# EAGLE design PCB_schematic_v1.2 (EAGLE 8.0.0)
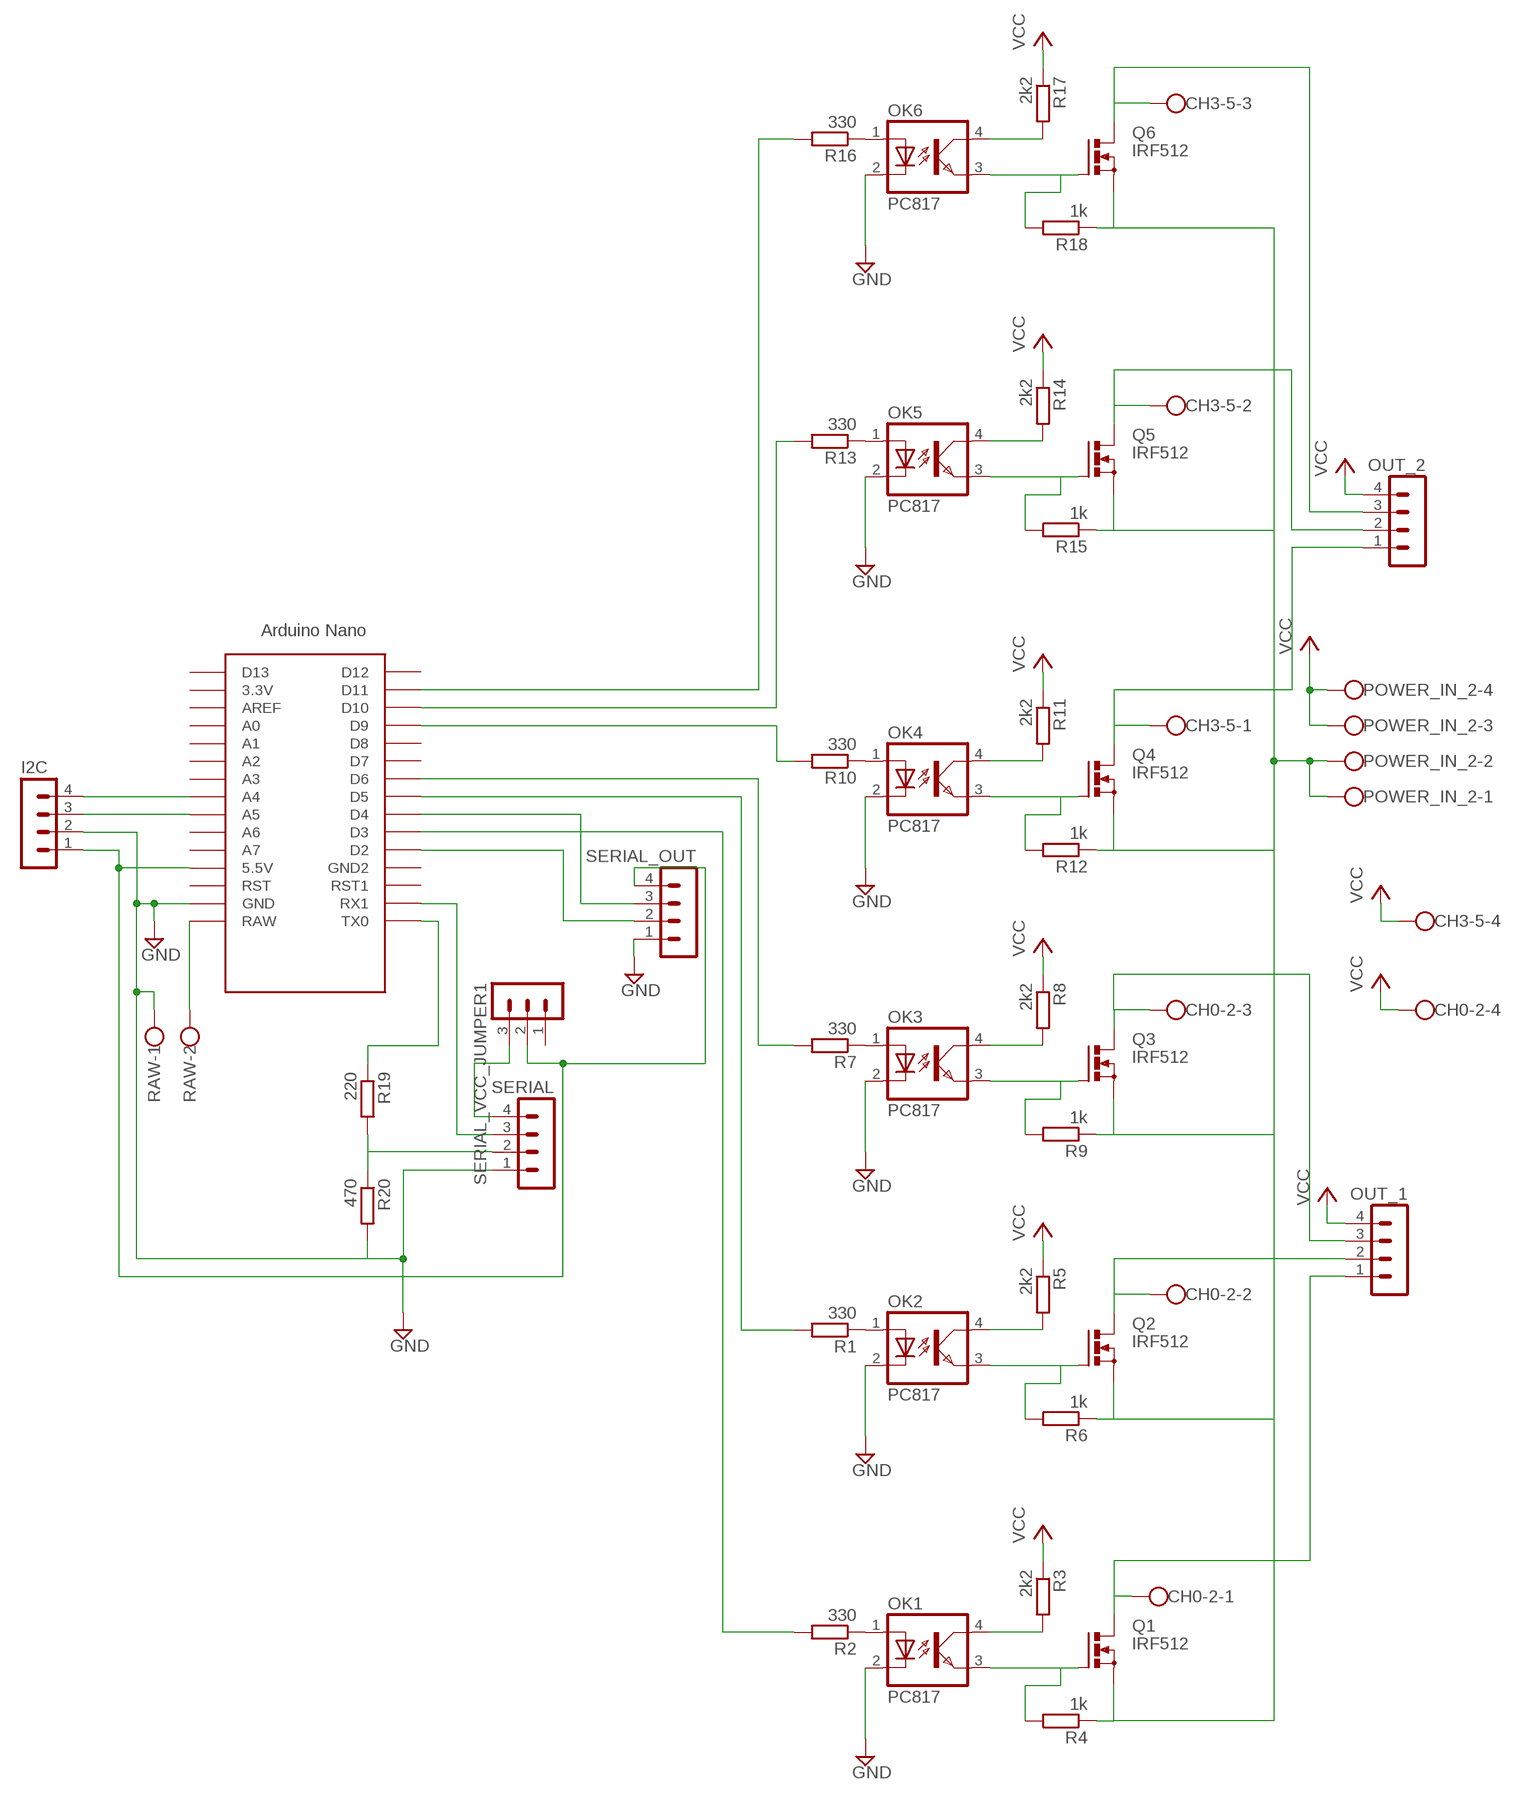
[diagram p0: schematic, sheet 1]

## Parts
CH0-2  W237-4  [W237-4]
CH3-5  W237-4  [W237-4]
I2C  MA04-1  [MA04-1]
OK1  PC817  [DIL04]
OK2  PC817  [DIL04]
OK3  PC817  [DIL04]
OK4  PC817  [DIL04]
OK5  PC817  [DIL04]
OK6  PC817  [DIL04]
OUT_1  MA04-1  [MA04-1]
OUT_2  MA04-1  [MA04-1]
POWER_IN_2  W237-4  [W237-4]
Q1  IRF512  [TO220BV]
Q2  IRF512  [TO220BV]
Q3  IRF512  [TO220BV]
Q4  IRF512  [TO220BV]
Q5  IRF512  [TO220BV]
Q6  IRF512  [TO220BV]
R1  330  R-EU_0207/10  [0207/10]
R2  330  R-EU_0207/10  [0207/10]
R3  2k2  R-EU_0207/10  [0207/10]
R4  1k  R-EU_0207/10  [0207/10]
R5  2k2  R-EU_0207/10  [0207/10]
R6  1k  R-EU_0207/10  [0207/10]
R7  330  R-EU_0207/10  [0207/10]
R8  2k2  R-EU_0207/10  [0207/10]
R9  1k  R-EU_0207/10  [0207/10]
R10  330  R-EU_0207/10  [0207/10]
R11  2k2  R-EU_0207/10  [0207/10]
R12  1k  R-EU_0207/10  [0207/10]
R13  330  R-EU_0207/10  [0207/10]
R14  2k2  R-EU_0207/10  [0207/10]
R15  1k  R-EU_0207/10  [0207/10]
R16  330  R-EU_0207/10  [0207/10]
R17  2k2  R-EU_0207/10  [0207/10]
R18  1k  R-EU_0207/10  [0207/10]
R19  220  R-EU_0207/10  [0207/10]
R20  470  R-EU_0207/10  [0207/10]
RAW  W237-102  [W237-102]
SERIAL  MA04-1  [MA04-1]
SERIAL_OUT  MA04-1  [MA04-1]
SERIAL_VCC_JUMPER1  MA03-1  [MA03-1]
U$1  NANO  [NANO]

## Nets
EXT_GND: POWER_IN_2.1 POWER_IN_2.2 Q1.S Q2.S Q3.S Q4.S Q5.S Q6.S R4.1 R6.1 R9.1 R12.1 R15.1 R18.1
EXT_VCC_12V: CH0-2.4 CH3-5.4 OUT_1.4 OUT_2.4 R3.1 R5.1 R8.1 R11.1 R14.1 R17.1 ; supply symbol labelled VCC
FET0_GATE: OK1.3(EMIT) Q1.G R4.2
FET0_GATE1: OK2.3(EMIT) Q2.G R6.2
FET0_GATE2: OK3.3(EMIT) Q3.G R9.2
FET0_GATE3: OK4.3(EMIT) Q4.G R12.2
FET0_GATE4: OK5.3(EMIT) Q5.G R15.2
FET0_GATE5: OK6.3(EMIT) Q6.G R18.2
GND: I2C.2 OK1.2(C) OK2.2(C) OK3.2(C) OK4.2(C) OK5.2(C) OK6.2(C) R20.2 RAW.1 SERIAL.1 SERIAL_OUT.1 U$1.GND
IC_PWM_OUT_0: R2.2 U$1.D3
IC_PWM_OUT_0_BASE: OK1.1(A) R2.1
IC_PWM_OUT_0_BASE1: OK2.1(A) R1.1
IC_PWM_OUT_0_BASE2: OK3.1(A) R7.1
IC_PWM_OUT_0_BASE3: OK4.1(A) R10.1
IC_PWM_OUT_0_BASE4: OK5.1(A) R13.1
IC_PWM_OUT_0_BASE5: OK6.1(A) R16.1
IC_PWM_OUT_1: R1.2 U$1.D5
IC_PWM_OUT_2: R7.2 U$1.D6
IC_PWM_OUT_3: R10.2 U$1.D9
IC_PWM_OUT_4: R13.2 U$1.D10
IC_PWM_OUT_5: R16.2 U$1.D11
IC_VCC_5V: I2C.1 SERIAL_OUT.4 SERIAL_VCC_JUMPER1.2 U$1.5V(5.5V)
N$1: OK1.4(COL) R3.2
N$3: OK2.4(COL) R5.2
N$5: OK3.4(COL) R8.2
N$7: OK4.4(COL) R11.2
N$9: OK5.4(COL) R14.2
N$11: OK6.4(COL) R17.2
N$28: SERIAL_OUT.3 U$1.D4
N$29: SERIAL_OUT.2 U$1.D2
OUTPUT_0: CH0-2.1 OUT_1.1 Q1.D
OUTPUT_1: CH0-2.2 OUT_1.2 Q2.D
OUTPUT_2: CH0-2.3 OUT_1.3 Q3.D
OUTPUT_3: CH3-5.1 OUT_2.1 Q4.D
OUTPUT_4: CH3-5.2 OUT_2.2 Q5.D
OUTPUT_5: CH3-5.3 OUT_2.3 Q6.D
RAW_INPUT: RAW.2 U$1.RAW
RX: SERIAL.3 U$1.RX1
SCL: I2C.3 U$1.A5
SDA: I2C.4 U$1.A4
SERIAL_VCC: SERIAL.4 SERIAL_VCC_JUMPER1.3
TX_3,3V: R19.2 R20.1 SERIAL.2
TX_5V: R19.1 U$1.TX0
VCC: POWER_IN_2.3 POWER_IN_2.4
Unconnected: SERIAL_VCC_JUMPER1.1 U$1.3.3V U$1.A0 U$1.A1 U$1.A2 U$1.A3 U$1.A6 U$1.A7 U$1.AREF U$1.D7 U$1.D8 U$1.D12 U$1.D13 U$1.GND1(GND2) U$1.ICSP1 U$1.ICSP2 U$1.ICSP3 U$1.ICSP4 U$1.ICSP5 U$1.ICSP6 U$1.RST U$1.RST1

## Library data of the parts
CH0-2 CH3-5 POWER_IN_2 = con-wago-500:W237-4: WAGO SCREW CLAMP; OC_FARNELL: unknown; OC_NEWARK: unknown
I2C OUT_1 OUT_2 SERIAL SERIAL_OUT = con-lstb:MA04-1: PIN HEADER; OC_FARNELL: unknown; OC_NEWARK: unknown
OK1-OK6 = optocoupler:PC817: SHARP OPTO COUPLER; MPN: PC817X4J000F; OC_FARNELL: 9707727; OC_NEWARK: 97K7059
Q1-Q6 = transistor-power:IRF512: N-CHANNEL MOS FET
R1-R20 = rcl:R-EU_: RESISTOR, European symbol
RAW = con-wago-500:W237-102: WAGO SCREW CLAMP; MPN: 237-102; OC_FARNELL: unknown; OC_NEWARK: 70K9898
SERIAL_VCC_JUMPER1 = con-lstb:MA03-1: PIN HEADER; OC_FARNELL: unknown; OC_NEWARK: unknown
U$1 = Arduino-clone:NANO: Arduino Nano

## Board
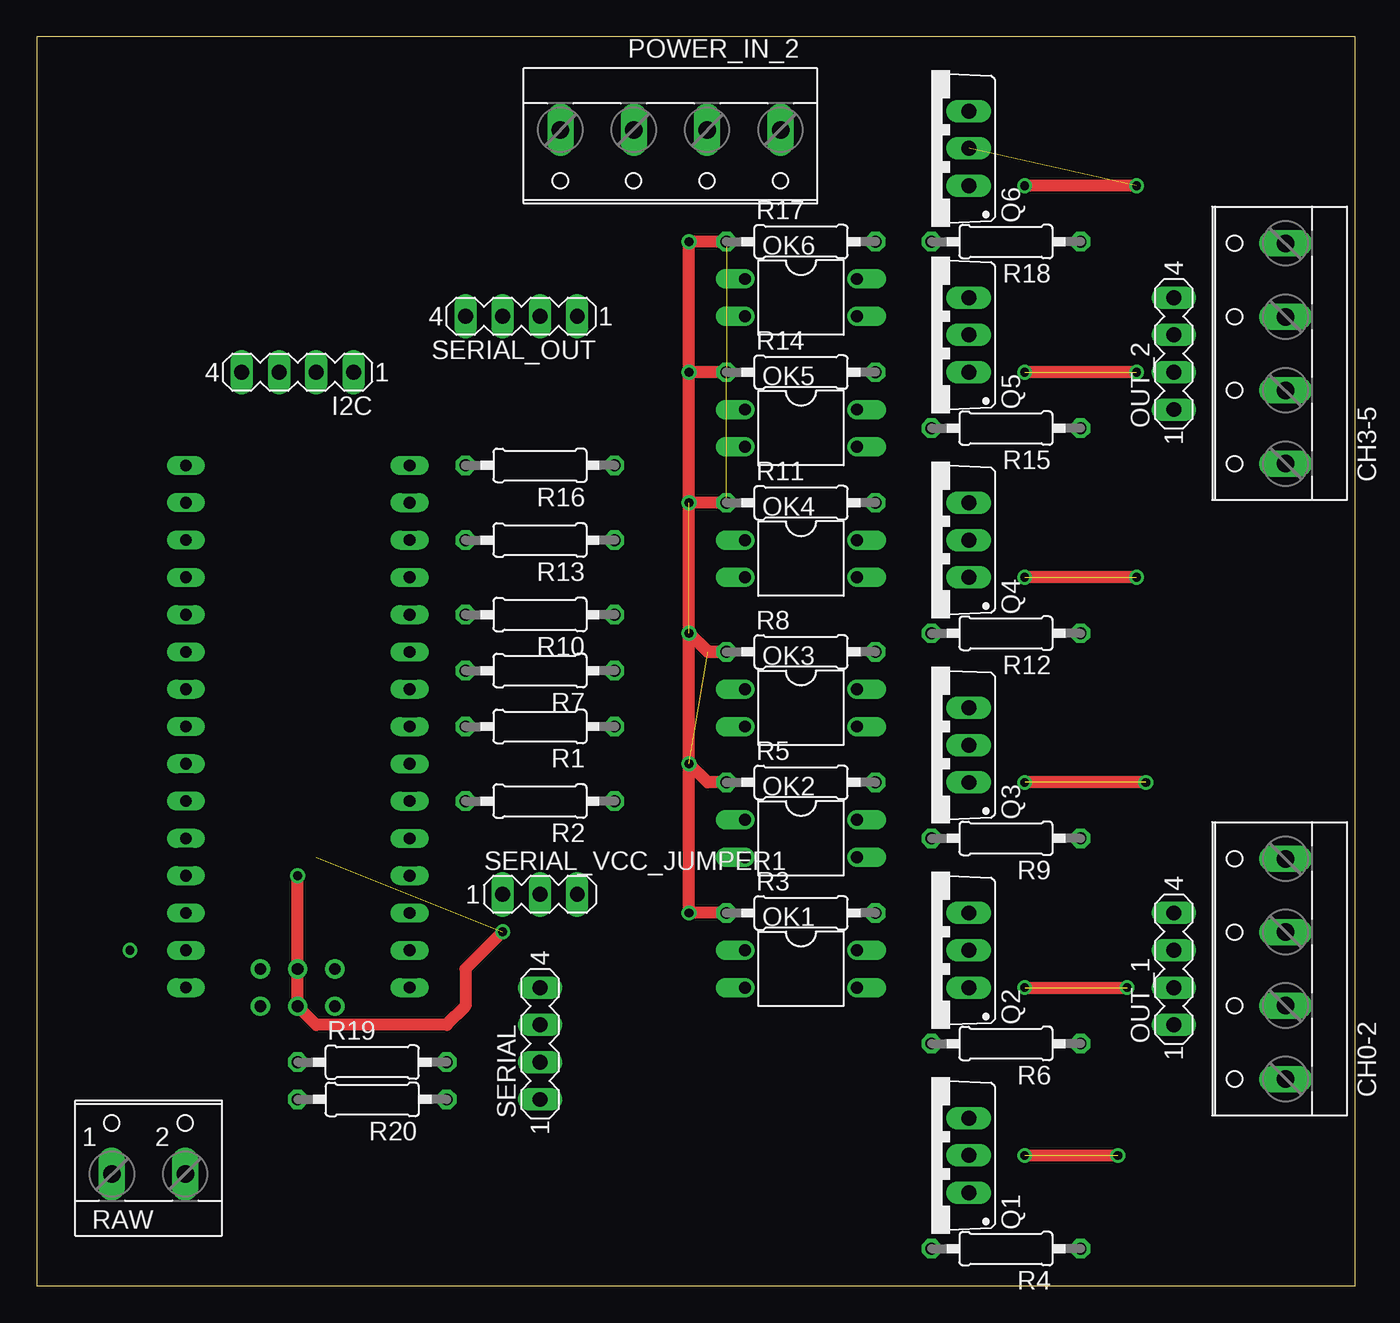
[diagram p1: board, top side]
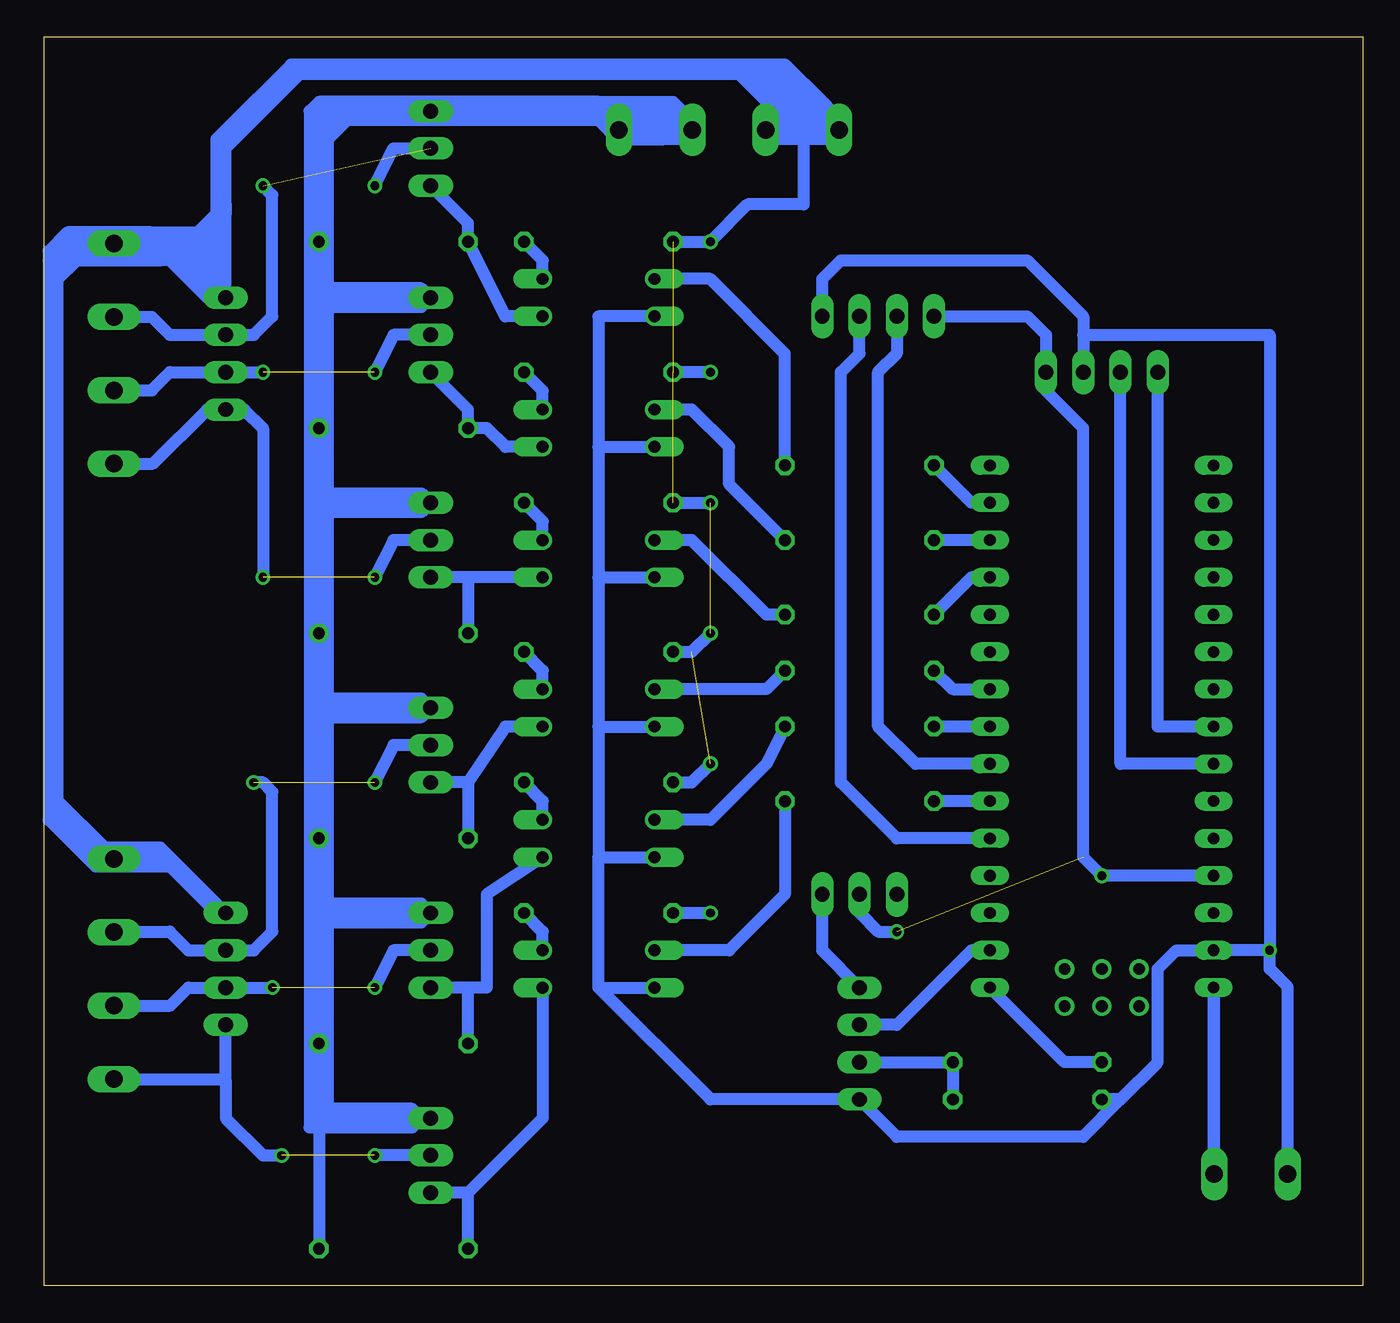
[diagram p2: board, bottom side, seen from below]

Size 89.84 x 85.08 mm. Coordinates in mm from the lower left corner, seen from the top.
Outline: 0,0 89.84,0 89.84,85.08 0,85.08 0,0
Copper layers (1*16): Top 0.035mm / dielectric 1.5mm / Bottom 0.035mm
Design rules "default": minimum track width 10mil, minimum drill 24mil, track to track 8mil, track to pad 8mil, pad to pad 8mil, via to via 8mil, smd to smd 8mil, copper to edge 40mil, drill to drill 8mil, minimum pad ring 10mil, minimum via ring 8mil, stop-mask expansion 4mil, vias tented up to drill 0mil, thermal gap 10mil

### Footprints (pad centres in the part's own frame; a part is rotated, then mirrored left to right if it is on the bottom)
W237-4 = drill 1.194 long: 1 -7.5,-1.27; 2 -2.5,-1.27; 3 2.5,-1.27; 4 7.5,-1.27
MA04-1 = drill 1.016 long: 1 -3.81,0; 2 -1.27,0; 3 1.27,0; 4 3.81,0
DIL04 = drill 0.813 offset: 1 -1.27,-3.81; 2 1.27,-3.81; 3 1.27,3.81; 4 -1.27,3.81
TO220BV = drill 1.016 long: D 0,-2.54; G -2.54,-2.54; S 2.54,-2.54
0207/10 = drill 0.813 octagon: 1 -5.08,0; 2 5.08,0
W237-102 = drill 1.194 long: 1 -2.5,-1.27; 2 2.5,-1.27
MA03-1 = drill 1.016 long: 1 -2.54,0; 2 0,0; 3 2.54,0
NANO = drill 0.8 long: 3.3V -10.16,24.13; 5V -10.16,-1.27; A0 -10.16,19.05; A1 -10.16,16.51; A2 -10.16,13.97; A3 -10.16,11.43; A4 -10.16,8.89; A5 -10.16,6.35; A6 -10.16,3.81; A7 -10.16,1.27; AREF -10.16,21.59; D2 5.08,1.27; D3 5.08,3.81; D4 5.08,6.35; D5 5.08,8.89; D6 5.08,11.43; D7 5.08,13.97; D8 5.08,16.51; D9 5.08,19.05; D10 5.08,21.59; D11 5.08,24.13; D12 5.08,26.67; D13 -10.16,26.67; GND -10.16,-6.35; GND1 5.08,-1.27; RAW -10.16,-8.89; RST -10.16,-3.81; RST1 5.08,-3.81; RX1 5.08,-6.35; TX0 5.08,-8.89 | drill 0.8: ICSP1 -5.08,-10.16; ICSP2 -5.08,-7.62; ICSP3 -2.54,-10.16; ICSP4 -2.54,-7.62; ICSP5 0,-10.16; ICSP6 0,-7.62

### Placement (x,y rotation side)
CH0-2  83.82,21.59 90 top
CH3-5  83.82,63.5 90 top
I2C  17.78,62.23 180 top
OK1  52.07,21.59 270 top
OK2  52.07,30.48 270 top
OK3  52.07,39.37 270 top
OK4  52.07,49.53 270 top
OK5  52.07,58.42 270 top
OK6  52.07,67.31 270 top
OUT_1  77.47,21.59 90 top
OUT_2  77.47,63.5 90 top
POWER_IN_2  43.18,77.47 180 top
Q1  60.96,8.89 90 top
Q2  60.96,22.86 90 top
Q3  60.96,36.83 90 top
Q4  60.96,50.8 90 top
Q5  60.96,64.77 90 top
Q6  60.96,77.47 90 top
R1  34.29,38.1 180 top
R2  34.29,33.02 180 top
R3  52.07,25.4 0 top
R4  66.04,2.54 180 top
R5  52.07,34.29 0 top
R6  66.04,16.51 180 top
R7  34.29,41.91 180 top
R8  52.07,43.18 0 top
R9  66.04,30.48 180 top
R10  34.29,45.72 180 top
R11  52.07,53.34 0 top
R12  66.04,44.45 180 top
R13  34.29,50.8 180 top
R14  52.07,62.23 0 top
R15  66.04,58.42 180 top
R16  34.29,55.88 180 top
R17  52.07,71.12 0 top
R18  66.04,71.12 180 top
R19  22.86,15.24 0 top
R20  22.86,12.7 180 top
RAW  7.62,8.89 0 top
SERIAL  34.29,16.51 90 top
SERIAL_OUT  33.02,66.04 180 top
SERIAL_VCC_JUMPER1  34.29,26.67 0 top
U$1  20.32,29.21 0 top

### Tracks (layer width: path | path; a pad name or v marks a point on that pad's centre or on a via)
EXT_GND
  Bottom 0.813: 71.12,11.43 R4.1 | 71.12,11.43 R6.1 71.12,25.4 | 71.12,25.4 R9.1 71.12,39.37 | 71.12,39.37 R12.1 | 71.12,53.34 R15.1 | 71.12,53.34 R12.1 | 71.12,66.67 R15.1 | 71.12,79.38 71.12,80.01 69.22,80.01 | 71.12,78.74 71.12,78.11 | 71.12,78.11 R18.1 71.12,67.31 | Q5.S 71.12,67.31 | Q4.S 71.12,53.34 | Q2.S 71.12,25.4 | Q1.S 64.14,11.43 | 64.14,11.43 71.12,11.43 | Q6.S 52.07,80.01 50.8,78.7 POWER_IN_2.2 POWER_IN_2.1 | Q6.S 69.22,80.01 | R15.1 R12.1 | Q3.S 71.12,39.37 | 69.22,79.38 52.07,79.38 50.8,78.11 50.16,78.11 | 69.22,79.38 70.48,79.38 | 70.48,79.38 71.12,78.74 | 71.12,78.74 71.12,79.38 | 71.12,79.38 70.48,79.38 | 50.16,78.11 50.16,78.74 52.07,80.64 | 52.07,80.64 71.12,80.64 71.75,80.01 71.75,10.79 64.77,10.79 64.14,11.43 | 64.14,11.43 64.77,12.06 70.48,12.06 70.48,24.77 | 70.48,26.04 70.48,38.73 | 70.48,40.01 70.48,52.7 | 70.48,53.98 70.48,78.11 69.22,79.38 | 70.48,52.7 64.14,52.7 Q4.S | 70.48,52.7 70.48,53.98 | 70.48,53.98 64.14,53.98 Q4.S | Q3.S 64.14,40.01 70.48,40.01 | 70.48,40.01 70.48,38.73 | 70.48,38.73 64.14,38.73 Q3.S | Q2.S 64.14,26.04 70.48,26.04 | 70.48,26.04 70.48,24.77 | 70.48,24.77 64.14,24.77 Q2.S | Q5.S 64.14,67.94 70.48,67.94 71.12,67.31 | 71.12,67.31 71.12,66.67 | 71.12,66.67 64.14,66.67 Q5.S | 71.12,78.11 69.22,80.01 | Q6.S 52.7,80.01 52.07,80.64 | 52.07,80.64 46.99,80.64 45.72,79.38 45.72,78.11 47.62,78.11 | 50.16,78.11 47.62,78.11 | 47.62,78.11 46.35,79.38 | 46.35,79.38 46.99,79.38 | 46.99,79.38 47.62,80.01 | 47.62,80.01 46.99,80.01 46.35,79.38 | 46.99,79.38 50.16,79.38 50.8,80.01 47.62,80.01
EXT_VCC_12V  (4 unrouted)
  Top 0.813: R14.1 44.45,62.23 | R17.1 44.45,71.12 | R11.1 44.45,53.34 | R5.1 45.72,34.29 44.45,35.56 44.45,25.4 R3.1 | R8.1 45.72,43.18 44.45,44.45
  Bottom 0.813: OUT_1.4 81.16,29.09 CH0-2.4 86.24,29.09 88.9,31.75 88.9,32.38 | 81.28,69.85 82.43,71 CH3-5.4 85.21,71.12 87.63,71.12 | 81.28,69.85 79.38,67.94 | 78.74,67.31 OUT_2.4 77.47,73.03 | R17.1 44.45,71.12 41.91,73.66 38.1,73.66 38.1,80.64 | R11.1 44.45,53.34 | R8.1 45.72,43.18 44.45,44.45 | R5.1 45.72,34.29 44.45,35.56 | R3.1 44.45,25.4 | 77.47,73.66 77.47,77.47 72.39,82.55 42.55,82.55 | 41.91,82.55 41.27,82.55 | 41.27,82.55 40.64,82.55 | 40.01,82.55 39.37,82.55 38.1,81.28 38.1,80.64 | 88.9,33.02 88.9,68.58 | 88.9,68.58 88.9,69.85 88.27,70.48 | 40.64,80.01 40.64,79.38 | 40.64,79.38 38.73,79.38 | 38.73,79.38 35.56,79.38 | 35.56,79.38 35.56,78.11 40.64,78.11 40.64,79.38 | 38.73,79.38 38.73,80.64 40.64,82.55 | 40.64,82.55 40.01,82.55 | 40.01,82.55 38.1,80.64 | 38.1,80.64 36.83,80.64 | 36.83,80.64 36.2,80.01 | 36.2,80.01 35.56,79.38 | 36.83,80.64 39.37,83.19 72.39,83.19 | 72.39,83.19 73.03,83.19 77.47,78.74 | 77.47,78.74 78.11,78.11 78.11,69.22 | 78.11,69.22 78.74,68.58 | 78.74,68.58 79.38,68.58 | 79.38,68.58 80.01,69.22 | 80.01,69.22 81.92,71.12 | 81.92,71.12 82.55,71.75 | 82.55,71.75 88.27,71.75 89.53,70.48 89.53,69.85 | 89.53,69.85 89.53,31.75 86.36,28.57 81.28,28.57 78.11,25.4 OUT_1.4 | OUT_1.4 81.92,29.84 85.72,29.84 88.9,33.02 | 88.9,33.02 88.9,32.38 | 88.9,32.38 85.72,29.21 | 88.27,70.48 87.63,71.12 | 87.63,71.12 88.27,71.12 89.53,69.85 | 89.53,69.85 87.63,69.85 | 87.63,69.85 81.92,69.85 | 81.28,69.85 81.92,69.85 | 81.92,69.85 82.55,70.48 88.27,70.48 | 79.38,68.58 79.38,67.94 | 79.38,67.94 78.74,67.31 | 78.74,67.31 78.11,67.94 78.11,68.58 | 78.11,69.22 78.11,68.58 | 78.11,68.58 78.74,67.94 | 88.9,68.58 87.63,69.85 | 82.55,71.75 79.38,71.75 77.47,73.66
  Bottom 0.813: 77.47,73.66 77.47,73.03 | 77.47,73.03 79.38,71.12 81.28,71.12 | 81.92,71.12 81.28,71.12 | 81.28,71.12 80.64,70.48 | 80.64,70.48 78.74,68.58 | 78.74,68.58 78.74,69.85 | 78.74,69.85 78.74,71.12 80.01,71.12 80.64,70.48 | 80.64,70.48 79.38,70.48 78.74,69.85 | 78.74,69.85 79.38,69.85 80.01,69.22 | 80.01,69.22 79.38,69.22 78.74,69.85 | 77.47,78.74 77.47,78.11 72.39,83.19 | 36.2,80.01 40.64,80.01 | 40.64,80.01 40.64,80.64 42.55,82.55 | 42.55,82.55 41.91,82.55 | 41.91,82.55 40.01,80.64 39.37,80.64 41.27,82.55
FET0_GATE
  Bottom 0.813: R4.2 60.96,6.35 | OK1.3 55.88,11.43 60.96,6.35 | 60.96,6.35 Q1.G
FET0_GATE1
  Bottom 0.813: R6.2 60.96,20.32 | OK2.3 59.69,26.67 59.69,20.32 60.96,20.32 | 60.96,20.32 Q2.G
FET0_GATE2
  Bottom 0.813: 60.96,34.29 Q3.G | OK3.3 58.42,38.1 60.96,34.29 | 60.96,34.29 R9.2
FET0_GATE3
  Bottom 0.813: 60.96,48.26 R12.2 | 60.96,48.26 Q4.G | OK4.3 60.96,48.26
FET0_GATE4
  Bottom 0.813: Q5.G 60.96,59.69 R15.2 59.69,58.42 58.42,57.15 OK5.3
FET0_GATE5
  Bottom 0.813: Q6.G 60.96,72.39 R18.2 58.42,66.04 OK6.3
GND  (via drill 0.6)
  Bottom 0.813: OK6.2 52.07,66.04 52.07,57.15 | 52.07,57.15 OK5.2 | 52.07,57.15 52.07,48.26 | 52.07,48.26 OK4.2 | 52.07,48.26 52.07,38.1 | 52.07,38.1 OK3.2 | 52.07,38.1 52.07,29.21 | 52.07,29.21 OK2.2 | 52.07,20.32 52.07,29.21 | 52.07,20.32 OK1.2 | 52.07,20.32 44.45,12.7 SERIAL.1 31.75,10.16 19.05,10.16 16.51,12.7 | 16.51,12.7 R20.2 | 16.51,12.7 13.97,15.24 13.97,21.59 12.7,22.86 U$1.GND v6.35,22.86 | 19.05,64.77 I2C.2 | 19.05,64.77 6.35,64.77 v6.35,22.86 | RAW.1 5.12,20.36 6.35,21.59 v6.35,22.86 | SERIAL_OUT.1 36.83,68.58 35.56,69.85 22.86,69.85 19.05,66.04 19.05,64.77
IC_PWM_OUT_0
  Bottom 0.813: U$1.D3 R2.2
IC_PWM_OUT_0_BASE
  Bottom 0.813: R2.1 39.37,26.67 43.18,22.86 OK1.1
IC_PWM_OUT_0_BASE1
  Bottom 0.813: R1.1 40.64,35.56 44.45,31.75 OK2.1
IC_PWM_OUT_0_BASE2
  Bottom 0.813: R7.1 40.64,40.64 OK3.1
IC_PWM_OUT_0_BASE3
  Bottom 0.813: R10.1 40.64,45.72 45.72,50.8 OK4.1
IC_PWM_OUT_0_BASE4
  Bottom 0.813: R13.1 43.18,54.61 43.18,57.15 45.72,59.69 OK5.1
IC_PWM_OUT_0_BASE5
  Bottom 0.813: R16.1 39.37,63.5 44.45,68.58 OK6.1
IC_PWM_OUT_1
  Bottom 0.813: U$1.D5 R1.2
IC_PWM_OUT_2
  Bottom 0.813: R7.2 27.94,40.64 U$1.D6
IC_PWM_OUT_3
  Bottom 0.813: U$1.D9 26.67,48.26 R10.2
IC_PWM_OUT_4
  Bottom 0.813: U$1.D10 R13.2
IC_PWM_OUT_5
  Bottom 0.813: U$1.D11 26.67,53.34 R16.2
IC_VCC_5V  (1 unrouted)
  Bottom 0.813: U$1.5V 17.78,27.94 19.05,29.21 19.05,58.42 21.59,60.96 I2C.1 21.59,64.77 22.86,66.04 SERIAL_OUT.4 | SERIAL_VCC_JUMPER1.2 34.29,25.4 33.02,24.13 31.75,24.13
N$1
  Bottom 0.813: OK1.4 55.88,24.13 R3.2
N$2  (via drill 0.6)
  other vias: 6.35,22.86
N$3
  Bottom 0.813: OK2.4 55.88,33.02 R5.2
N$4  (via drill 0.6)
  Top 0.813: v31.75,24.13 29.21,21.59 29.21,19.05 27.94,17.78 19.05,17.78 17.78,19.05 17.78,27.94
N$5
  Bottom 0.813: OK3.4 55.88,41.91 R8.2
N$6  (via drill 0.6)
  other vias: 17.78,27.94
N$7
  Bottom 0.813: OK4.4 55.88,52.07 R11.2
N$8  (via drill 0.6)
  Top 0.813: v67.31,8.89 73.66,8.89
N$9
  Bottom 0.813: OK5.4 55.88,60.96 R14.2
N$10  (via drill 0.6)
  Top 0.813: v67.31,20.32 74.3,20.32
N$11
  Bottom 0.813: OK6.4 55.88,69.85 R17.2
N$12  (via drill 0.6)  (1 unrouted)
  other vias: 67.31,34.29
N$13  (via drill 0.6)
  other vias: 67.31,48.26
N$14  (via drill 0.6)
  other vias: 67.31,62.23
N$15  (via drill 0.6)
  Bottom 0.813: v67.31,74.93 66.04,77.47 63.5,77.47
N$16  (via drill 0.6)
  Top 0.813: v74.93,74.93 67.31,74.93
N$17  (via drill 0.6)
  Top 0.813: v74.93,62.23 67.31,62.23
N$18  (via drill 0.6)
  Top 0.813: v74.93,48.26 67.31,48.26
N$19  (via drill 0.6)
  Top 0.813: v75.56,34.29 67.31,34.29
N$20  (via drill 0.6)
  other vias: 74.3,20.32
N$21  (via drill 0.6)
  other vias: 73.66,8.89
N$22  (via drill 0.6)
  Top 0.813: v44.45,25.4 44.45,53.34
N$23  (via drill 0.6)
  Top 0.813: 46.99,43.18 45.72,43.18 44.45,44.45 v44.45,35.56
N$24  (via drill 0.6)
  other vias: 44.45,44.45
N$25  (via drill 0.6)
  other vias: 44.45,53.34
N$26  (via drill 0.6)
  Top 0.813: 44.45,53.34 v44.45,62.23 44.45,71.12
  Bottom 0.813: v44.45,62.23 46.99,62.23
N$27  (via drill 0.6)
  other vias: 44.45,71.12
N$28
  Bottom 0.813: U$1.D4 30.48,35.56 33.02,38.1 33.02,62.23 31.75,63.5 SERIAL_OUT.3
N$29
  Bottom 0.813: U$1.D2 31.75,30.48 35.56,34.29 35.56,62.23 34.29,63.5 SERIAL_OUT.2
OUTPUT_0  (1 unrouted)
  Bottom 0.813: 77.47,13.97 OUT_1.1 | 77.47,13.97 77.47,11.43 74.93,8.89 73.66,8.89 | CH0-2.1 77.59,14.09 77.47,13.97 | Q1.D 67.31,8.89
OUTPUT_1  (1 unrouted)
  Bottom 0.813: 74.3,20.32 OUT_1.2 80.01,20.32 81.24,19.09 CH0-2.2 | Q2.D 66.04,22.86 67.31,20.32
OUTPUT_2  (1 unrouted)
  Bottom 0.813: Q3.D 66.04,36.83 67.31,34.29 | CH0-2.3 85.05,24.13 81.28,24.13 80.01,22.86 OUT_1.3 75.56,22.86 74.3,24.13 74.3,33.66 74.93,34.29 75.56,34.29
OUTPUT_3  (1 unrouted)
  Bottom 0.813: Q4.D 66.04,50.8 67.31,48.26 | 74.93,48.26 74.93,58.42 76.2,59.69 OUT_2.1 78.74,59.69 82.43,56 CH3-5.1
OUTPUT_4  (1 unrouted)
  Bottom 0.813: Q5.D 66.04,64.77 67.31,62.23 | CH3-5.2 82.51,61 81.28,62.23 OUT_2.2 74.93,62.23
OUTPUT_5  (1 unrouted)
  Bottom 0.813: CH3-5.3 82.51,66 81.28,64.77 OUT_2.3 75.56,64.77 74.3,66.04 74.3,74.3 74.93,74.93
RAW_INPUT
  Bottom 0.813: 10.16,7.62 U$1.RAW 10.16,7.66 RAW.2
RX
  Bottom 0.813: U$1.RX1 26.67,22.86 31.75,17.78 SERIAL.3
SCL
  Bottom 0.813: U$1.A5 16.51,35.56 I2C.3
SDA
  Bottom 0.813: U$1.A4 13.97,38.1 I2C.4
SERIAL_VCC
  Bottom 0.813: SERIAL.4 36.83,22.86 SERIAL_VCC_JUMPER1.3
TX_3,3V
  Bottom 0.813: R20.1 R19.2 SERIAL.2
TX_5V
  Bottom 0.813: R19.1 20.32,15.24 U$1.TX0
VCC
  Bottom 0.813: 38.1,78.74 POWER_IN_2.3 38.1,78.74 | 38.1,78.74 POWER_IN_2.4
